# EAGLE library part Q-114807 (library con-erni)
Male Connector SMC-Q 68 contacts Standard Assembly Height Source: http://www.erni.com/DB/PDF-Drawing/SMC/114807.pdf
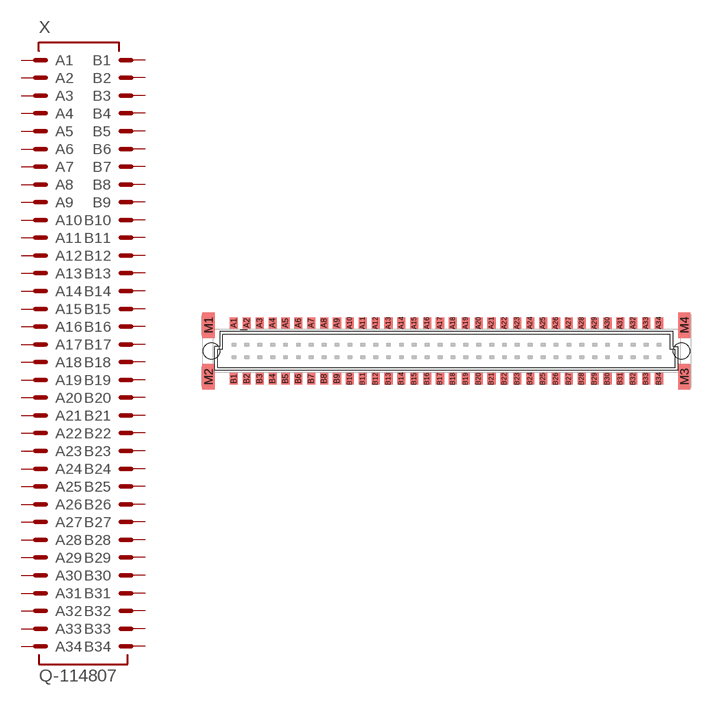
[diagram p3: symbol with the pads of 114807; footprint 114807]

Designator prefix X

## Q-114807 (OC_FARNELL: unknown; OC_NEWARK: unknown)  [114807]
A1  A1  pas
A2  A2  pas
A3  A3  pas
A4  A4  pas
A5  A5  pas
A6  A6  pas
A7  A7  pas
A8  A8  pas
A9  A9  pas
A10  A10  pas
A11  A11  pas
A12  A12  pas
A13  A13  pas
A14  A14  pas
A15  A15  pas
A16  A16  pas
A17  A17  pas
A18  A18  pas
A19  A19  pas
A20  A20  pas
A21  A21  pas
A22  A22  pas
A23  A23  pas
A24  A24  pas
A25  A25  pas
A26  A26  pas
A27  A27  pas
A28  A28  pas
A29  A29  pas
A30  A30  pas
A31  A31  pas
A32  A32  pas
A33  A33  pas
A34  A34  pas
B1  B1  pas
B2  B2  pas
B3  B3  pas
B4  B4  pas
B5  B5  pas
B6  B6  pas
B7  B7  pas
B8  B8  pas
B9  B9  pas
B10  B10  pas
B11  B11  pas
B12  B12  pas
B13  B13  pas
B14  B14  pas
B15  B15  pas
B16  B16  pas
B17  B17  pas
B18  B18  pas
B19  B19  pas
B20  B20  pas
B21  B21  pas
B22  B22  pas
B23  B23  pas
B24  B24  pas
B25  B25  pas
B26  B26  pas
B27  B27  pas
B28  B28  pas
B29  B29  pas
B30  B30  pas
B31  B31  pas
B32  B32  pas
B33  B33  pas
B34  B34  pas

## Footprint 114807 (pad centres in mm)
Male Connector SMC-Q 68 contacts Standard Assembly Height Source: http://www.erni.com/DB/PDF-Drawing/SMC/114807.pdf
smd 0.8 x 1.1: A1 -20.955,2.765; A2 -19.685,2.765; A3 -18.415,2.765; A4 -17.145,2.765; A5 -15.875,2.765; A6 -14.605,2.765; A7 -13.335,2.765; A8 -12.065,2.765; A9 -10.795,2.765; A10 -9.525,2.765; A11 -8.255,2.765; A12 -6.985,2.765; A13 -5.715,2.765; A14 -4.445,2.765; A15 -3.175,2.765; A16 -1.905,2.765; A17 -0.635,2.765; A18 0.635,2.765; A19 1.905,2.765; A20 3.175,2.765; A21 4.445,2.765; A22 5.715,2.765; A23 6.985,2.765; A24 8.255,2.765; A25 9.525,2.765; A26 10.795,2.765; A27 12.065,2.765; A28 13.335,2.765; A29 14.605,2.765; A30 15.875,2.765; A31 17.145,2.765; A32 18.415,2.765; A33 19.685,2.765; A34 20.955,2.765; B1 -20.955,-2.74; B2 -19.685,-2.74; B3 -18.415,-2.74; B4 -17.145,-2.74; B5 -15.875,-2.74; B6 -14.605,-2.74; B7 -13.335,-2.74; B8 -12.065,-2.74; B9 -10.795,-2.74; B10 -9.525,-2.74; B11 -8.255,-2.74; B12 -6.985,-2.74; B13 -5.715,-2.74; B14 -4.445,-2.74; B15 -3.175,-2.74; B16 -1.905,-2.74; B17 -0.635,-2.74; B18 0.635,-2.74; B19 1.905,-2.74; B20 3.175,-2.74; B21 4.445,-2.74; B22 5.715,-2.74; B23 6.985,-2.74; B24 8.255,-2.74; B25 9.525,-2.74; B26 10.795,-2.74; B27 12.065,-2.74; B28 13.335,-2.74; B29 14.605,-2.74; B30 15.875,-2.74; B31 17.145,-2.74; B32 18.415,-2.74; B33 19.685,-2.74; B34 20.955,-2.74
smd 1.2 x 2.5: M1 -23.46,2.55; M2 -23.46,-2.55; M3 23.46,-2.55; M4 23.46,2.55
hole 1.6 at -23.165,0
hole 1.6 at 23.165,0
